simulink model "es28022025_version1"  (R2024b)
settings: Solver=FixedStepAuto  StartTime=0.0  StopTime=5  FixedStep=0.005  RelTol=1e-3
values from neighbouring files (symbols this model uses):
  a = 0.5    [scriptsimulink28022025.m]
  xzero = 1    [scriptsimulink28022025.m]
  yzero = 2    [scriptsimulink28022025.m]
  yzerodot = -1    [scriptsimulink28022025.m]

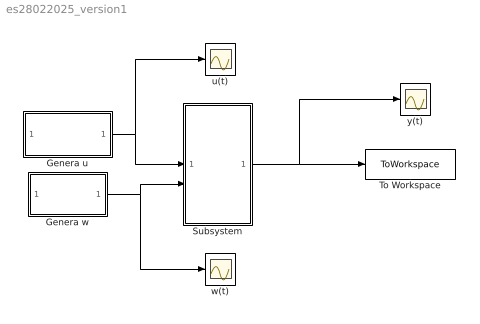
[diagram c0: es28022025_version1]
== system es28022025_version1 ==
  Genera u : Subsystem
  Genera w : Subsystem
  Subsystem : Subsystem
  To Workspace : ToWorkspace  VariableName=y  SaveFormat=Timeseries  SampleTime=-1
  u(t) : Scope
  w(t) : Scope
  y(t) : Scope
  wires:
  Genera u/1(u) -> u(t)/1, Subsystem/1(u)
  Genera w/1(w) -> w(t)/1, Subsystem/2(w)
  Subsystem/1(y) -> y(t)/1, To Workspace/1

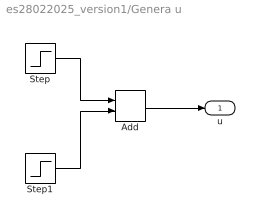
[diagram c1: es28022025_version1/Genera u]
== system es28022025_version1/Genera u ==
  Add : Sum
  Step : Step  Time=2  Before=2  After=6  SampleTime=0
  Step1 : Step  Time=3  After=-4  SampleTime=0
  u : Outport
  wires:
  Step/1 -> Add/1
  Step1/1 -> Add/2
  Add/1 -> u/1

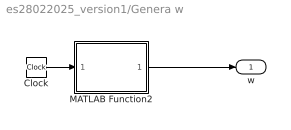
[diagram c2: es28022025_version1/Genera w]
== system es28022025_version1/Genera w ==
  Clock : Clock
  MATLAB Function2 : MATLAB Function  TreatAsAtomicUnit=on
  w : Outport
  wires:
  MATLAB Function2/1(w) -> w/1
  Clock/1 -> MATLAB Function2/1(t)

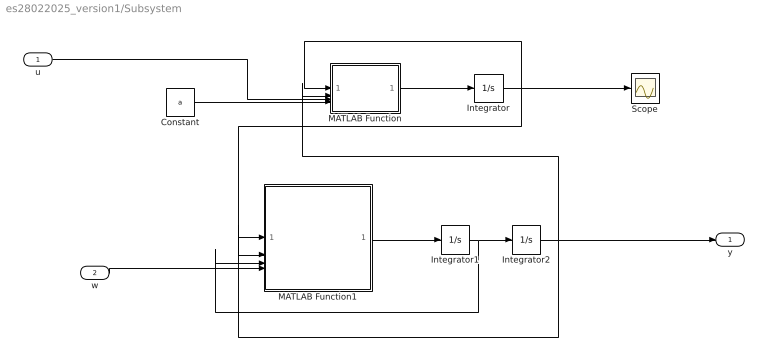
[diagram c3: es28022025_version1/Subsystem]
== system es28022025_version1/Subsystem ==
  u : Inport
  w : Inport  Port=2
  Constant : Constant  Value=a
  Integrator : Integrator  InitialCondition=xzero
  Integrator1 : Integrator  InitialCondition=yzerodot
  Integrator2 : Integrator  InitialCondition=yzero
  MATLAB Function : MATLAB Function  TreatAsAtomicUnit=on
  MATLAB Function1 : MATLAB Function  TreatAsAtomicUnit=on
  Scope : Scope
  y : Outport
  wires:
  Integrator1/1 -> MATLAB Function1/3(ydot), Integrator2/1
  w/1 -> MATLAB Function1/4(w)
  MATLAB Function1/1(yddot) -> Integrator1/1
  Integrator2/1 -> MATLAB Function1/2(y), y/1, MATLAB Function/2(y)
  Integrator/1 -> Scope/1, MATLAB Function/1(x), MATLAB Function1/1(x)
  MATLAB Function/1(xdot) -> Integrator/1
  Constant/1 -> MATLAB Function/4(a)
  u/1 -> MATLAB Function/3(u)

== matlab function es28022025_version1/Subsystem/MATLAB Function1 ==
function yddot = fcn(x,y,ydot,w)

yddot=-0.1*ydot*abs(ydot)-x*y+w/2;

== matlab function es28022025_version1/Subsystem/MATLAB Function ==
function xdot = fcn(x,y,u,a)

xdot=-a*x^3/4-(1/2)*(1/(abs(x)+1))+x*sin(2*x)/4-(sin(y))^2/4+u;

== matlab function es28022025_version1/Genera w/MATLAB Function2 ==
function w = fcn(t)

w=8*sin(3*t)*cos(10*t+1);
